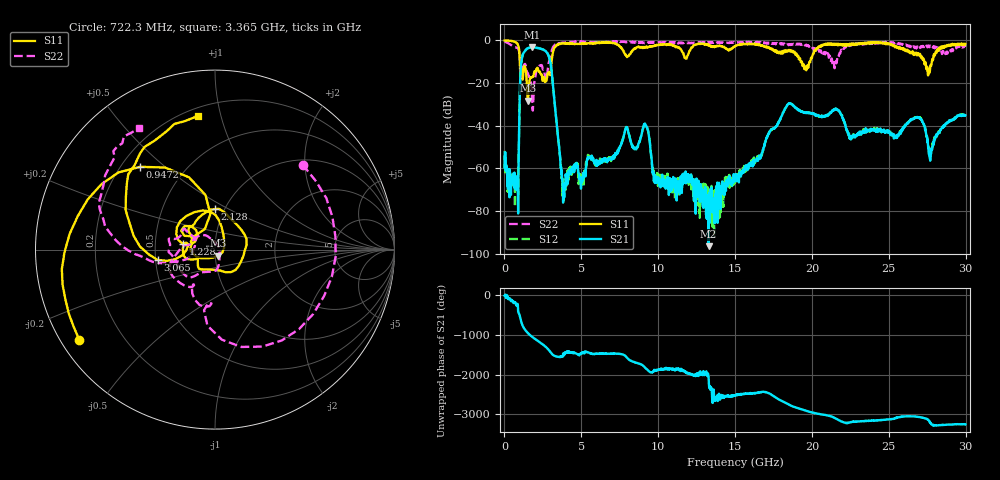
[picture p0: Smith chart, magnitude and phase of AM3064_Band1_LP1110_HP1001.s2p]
# Hz S DB R 50.0
!freq dBS11 angS11 dBS21 angS21 dBS12 angS12 dBS22 angS22
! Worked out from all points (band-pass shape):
!   1600 points, 10 MHz to 29.98 GHz, reference 50 ohm
!   highest |S21| = -3.23 dB at 1.791 GHz (marker M1); lowest = -96.5 dB at 13.28 GHz (marker M2)
!   |S21| within 3 dB of the highest: 1.217 GHz to 2.807 GHz (1.59 GHz wide, 79 % of centre)
!   lowest |S11| = -28.2 dB at 1.528 GHz (marker M3), VSWR 1.08, Z = 51.7 - j3.55 ohm
!   |S11| at or under -10 dB: 1.002 GHz to 3.062 GHz (2.06 GHz wide, 101 % of centre); 19.34 GHz to 19.89 GHz (542.7 MHz wide, 2.77 % of centre); 27.3 GHz to 27.8 GHz (497.2 MHz wide, 1.8 % of centre)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
!   |S22| runs from -32.9 to -0.4 dB; largest |S21 - S12| = 0.011
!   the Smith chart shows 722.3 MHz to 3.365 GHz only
!   S11 on the Smith chart (normalised r, x): 722.3 MHz: 0.05, -0.30; 947.2 MHz: 0.28, +0.42; 1.228 GHz: 0.70, +0.04; 2.128 GHz: 0.90, +0.43; 3.065 GHz: 0.51, -0.07; 3.365 GHz: 0.25, +0.85
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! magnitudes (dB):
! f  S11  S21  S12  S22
! 10 MHz  -0.1  -54.5  -51.8  -0.4
! 722.3 MHz  -0.8  -67.0  -66.5  -3.3
! 947.2 MHz  -4.1  -43.8  -43.6  -5.0
! 1.228 GHz  -14.9  -6.1  -6.0  -12.3
! 1.528 GHz  -28.2  -3.7  -3.6  -15.6
! 1.791 GHz  -17.2  -3.2  -3.2  -26.3
! 2.128 GHz  -12.9  -3.6  -3.5  -13.1
! 3.065 GHz  -9.8  -14.4  -14.3  -5.1
! 3.365 GHz  -2.5  -36.7  -36.8  -1.9
! 3.871 GHz  -1.3  -71.8  -71.4  -1.1
! 5.015 GHz  -1.4  -66.7  -63.3  -0.6
! 9.157 GHz  -3.4  -39.4  -39.2  -1.2
! 10 GHz  -2.2  -64.5  -65.9  -0.9
! 13.28 GHz  -2.6  -96.5  -72.5  -1.2
! 15 GHz  -2.7  -64.4  -64.7  -1.2
! 18.45 GHz  -5.1  -29.9  -29.7  -2.0
! 19.99 GHz  -8.3  -34.3  -34.2  -3.0
! 21.47 GHz  -1.8  -32.4  -32.4  -13.0
! 25 GHz  -1.4  -43.1  -42.9  -1.2
! 26.94 GHz  -6.5  -36.4  -36.4  -3.3
! 27.71 GHz  -11.5  -55.4  -51.3  -2.6
! 29.98 GHz  -1.7  -35.1  -35.2  -2.9
